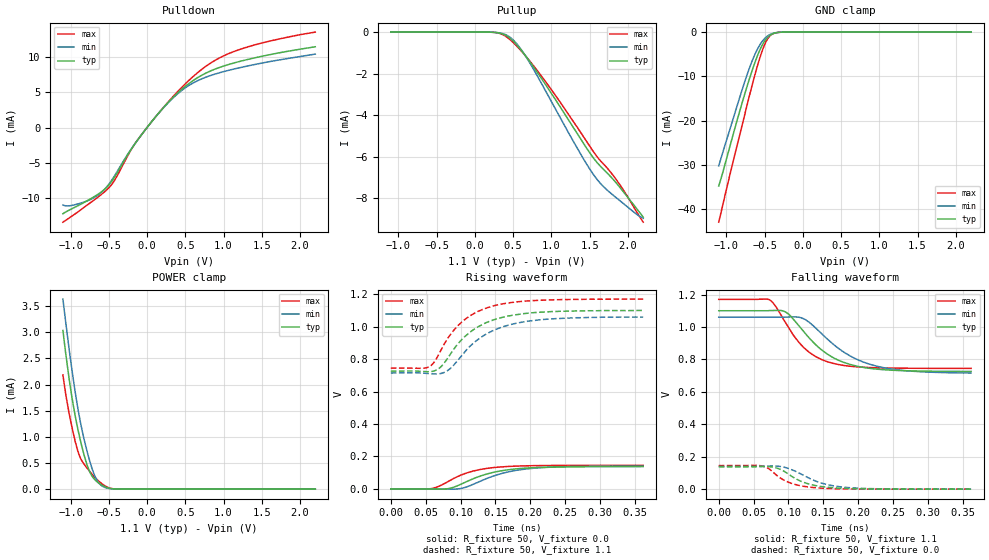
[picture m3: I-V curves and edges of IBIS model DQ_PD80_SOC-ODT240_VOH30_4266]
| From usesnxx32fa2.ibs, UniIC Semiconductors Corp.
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| DQ_PD80_SOC-ODT240_VOH30_4266
| (80 Ohm Pulldown, 240 Ohm System ODT Setting, VOH=VDDQ/3.0, 3200-4266Mbps)
[Model]   DQ_PD80_SOC-ODT240_VOH30_4266
Model_type   I/O
Vinl = 123.333mV
Vinh = 243.333mV
Vmeas = 183.333mV
Vref = 0.0mV
Cref = 0.0pF
Rref = 240.000Ohm
|   typ   min   max
|C_comp   0.834pF   0.784pF   0.884pF
C_comp_pullup   0.4170pF   0.3920pF   0.4420pF
C_comp_pulldown   0.4170pF   0.3920pF   0.4420pF
| Note: C_comp changes when the ODT circuit is enabled.
[Model Spec]
| Input threshold voltage corners
Vinl   0.1233V   0.1167V   0.1350V
Vinh   0.2433V   0.2367V   0.2550V
| Measurement voltage corners
Vmeas   0.1833V   0.1767V   0.1950V
| Timing spec test load voltage corners
Vref   0.0000V   0.0000V   0.0000V
| Dynamic Overshoot Parameters from LPDDR4 Specification
D_overshoot_ampl_h   0.30   NA   NA
D_overshoot_ampl_l   0.30   NA   NA
D_overshoot_area_h   0.1n   NA   NA
D_overshoot_area_l   0.1n   NA   NA
[Voltage Range]   1.1000V   1.0600V   1.1700V
[Pullup Reference]   1.1000V   1.0600V   1.1700V
| Junction Temperature (Ambient temp is 35C typ 95C min -40C max)
[Temperature Range]   50.0   110.0   -40.0
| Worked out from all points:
|   slope of the pulldown table from 0 to 0.165 V, typ, clamps not added: 74.6 ohm
|   slope of the pullup table from 0 to 0.165 V, typ, clamps not added: 79 kohm
|   GND clamp passes 1 mA (typ) near -0.45 V on its own axis
|   POWER clamp passes 1 mA (typ) near -0.88 V on its own axis
|   rising waveform, R_fixture 50, V_fixture 0.0: 20-80 % time 56.4ps typ, 58.8ps min, 49.1ps max; typ from 0 V to 0.137 V
|   falling waveform, R_fixture 50, V_fixture 1.1: 20-80 % time 57ps typ, 67.1ps min, 46.6ps max; typ from 1.1 V to 0.726 V
|   rising waveform, R_fixture 50, V_fixture 1.1: 20-80 % time 56.3ps typ, 60.5ps min, 52.1ps max; typ from 0.726 V to 1.1 V
|   falling waveform, R_fixture 50, V_fixture 0.0: 20-80 % time 39.1ps typ, 46.6ps min, 34.6ps max; typ from 0.137 V to 0 V
[Pulldown]
|   Voltage   I(typ)   I(min)   I(max)
-1.1V     -12.26mA   -11.01mA   -13.46mA
-1.014V   -11.72mA   -11.13mA   -12.83mA
-829.4mV  -10.7mA    -10.62mA   -11.4mA
-585.2mV  -9.054mA   -9.117mA   -9.415mA
-453.2mV  -7.519mA   -7.349mA   -7.968mA
-152.9mV  -2.228mA   -2.23mA    -2.227mA
203.5mV   2.691mA    2.665mA    2.709mA
467.5mV   5.553mA    5.379mA    5.855mA
734.8mV   7.541mA    7.005mA    8.425mA
955.9mV   8.569mA    7.808mA    9.942mA
1.25V     9.498mA    8.593mA    11.23mA
2.2V      11.48mA    10.44mA    13.57mA
[GND Clamp]
|   Voltage   I(typ)   I(min)   I(max)
-1.1V     -34.74mA   -30.21mA   -42.91mA
-1.05V    -31.86mA   -27.33mA   -39.27mA
-944.9mV  -25.23mA   -21.44mA   -31.55mA
-799.7mV  -16.31mA   -13.32mA   -21.42mA
-667.7mV  -8.907mA   -6.722mA   -12.29mA
-591.8mV  -5.255mA   -3.789mA   -7.492mA
-525.8mV  -2.77mA    -1.975mA   -3.963mA
-469.7mV  -1.356mA   -986.5uA   -1.787mA
-416.9mV  -598.6uA   -440.6uA   -664.6uA
-354.2mV  -179.4uA   -134.6uA   -160.3uA
-248.6mV  -12.13uA   -10.94uA   -7.108uA
2.2V      0A         0A         0A
[Pullup]
|   Voltage   I(typ)   I(min)   I(max)
-1.1V     1.046uA    1.612uA    471.3nA
236.5mV   -8.648uA   -8.621uA   -9.171uA
345.4mV   -66.92uA   -55.08uA   -92.21uA
454.3mV   -284.8uA   -236.7uA   -349.7uA
569.8mV   -713.8uA   -668.3uA   -763.3uA
695.2mV   -1.311mA   -1.351mA   -1.297mA
1.052V    -3.249mA   -3.698mA   -3.047mA
1.375V    -5.105mA   -5.833mA   -4.795mA
1.566V    -6.147mA   -6.95mA    -5.851mA
1.675V    -6.593mA   -7.426mA   -6.335mA
1.887V    -7.444mA   -8.098mA   -7.311mA
2.2V      -8.921mA   -8.97mA    -9.16mA
[POWER Clamp]
|   Voltage   I(typ)   I(min)   I(max)
-1.1V     3.033mA    3.633mA    2.184mA
-1.044V   2.381mA    2.967mA    1.653mA
-981.2mV  1.753mA    2.276mA    1.183mA
-911.9mV  1.201mA    1.61mA     764.6uA
-855.8mV  837.8uA    1.172mA    552.1uA
-796.4mV  521.2uA    794.7uA    427.2uA
-743.6mV  315.8uA    510.8uA    330.1uA
-671mV    164.5uA    216uA      210.1uA
-598.4mV  83.64uA    71.96uA    113uA
-492.8mV  18.89uA    11.54uA    24.03uA
-387.2mV  1.892uA    1.295uA    1.644uA
2.2V      0A         0A         0A
[Ramp]
|   typ   min   max
| 20% - 80%
dV/dt_r   82.33m/56.44p   84.05m/58.84p   87.12m/49.14p
dV/dt_f   224.45m/56.99p   206.39m/67.10p   255.14m/46.63p
| 25% - 75%
|dV/dt_r   68.61m/44.91p   70.04m/46.91p   72.60m/38.97p
|dV/dt_f   187.04m/45.37p   171.99m/53.48p   212.61m/37.05p
R_load = 50
[Rising Waveform]
R_fixture = 50
V_fixture = 0.0
|   Time   V(typ)   V(min)   V(max)
0s        121.8uV    91.42uV    94.29uV
57ps      -334uV     219.7uV    1.056mV
69ps      -1.57mV    -509.4uV   16.14mV
82ps      1.431mV    -1.454mV   45.18mV
106ps     39.55mV    8.234mV    93.91mV
128ps     78.59mV    46.74mV    119.3mV
151ps     105.4mV    84.79mV    132.9mV
180ps     123.4mV    114.3mV    140.5mV
215ps     132.5mV    130.7mV    143.7mV
362ps     137.3mV    140.2mV    145.3mV
[Falling Waveform]
R_fixture   = 50
V_fixture   = 1.1
V_fixture_min = 1.06
V_fixture_max = 1.17
|   Time   V(typ)   V(min)   V(max)
0s        1.1V       1.06V      1.17V
73ps      1.101V     1.06V      1.167V
83ps      1.102V     1.06V      1.119V
96ps      1.092V     1.061V     1.024V
120ps     981.4mV    1.054V     881.6mV
140ps     886.9mV    989.7mV    815.1mV
163ps     813.7mV    898mV      776.6mV
194ps     762.5mV    808.7mV    755.6mV
235ps     737mV      750.3mV    747.4mV
362ps     725.9mV    716mV      744.8mV
[Rising Waveform]
R_fixture   = 50
V_fixture   = 1.1
V_fixture_min = 1.06
V_fixture_max = 1.17
|   Time   V(typ)   V(min)   V(max)
0s        725.5mV    714.2mV    744.7mV
56ps      722.4mV    710.1mV    755.3mV
63ps      728.2mV    708.3mV    786.1mV
72ps      753.3mV    711.5mV    856.1mV
84ps      821.6mV    737.3mV    942.6mV
96ps      892.6mV    792.1mV    1.005V
120ps     985.4mV    904mV      1.083V
148ps     1.043V     978.2mV    1.129V
215ps     1.089V     1.043V     1.163V
362ps     1.1V       1.059V     1.17V
[Falling Waveform]
R_fixture = 50
V_fixture = 0.0
|   Time   V(typ)   V(min)   V(max)
0s        137.5mV    140.4mV    145.3mV
59ps      139.2mV    141.2mV    145.2mV
70ps      139.3mV    143mV      130.7mV
79ps      134.8mV    143.4mV    100.6mV
102ps     86.84mV    124.7mV    39.43mV
117ps     50.47mV    95.84mV    21.48mV
135ps     25.72mV    57.07mV    10.37mV
160ps     10.12mV    24.2mV     3.843mV
194ps     2.955mV    7.425mV    1.053mV
362ps     195.5uV    217.2uV    117.7uV
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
